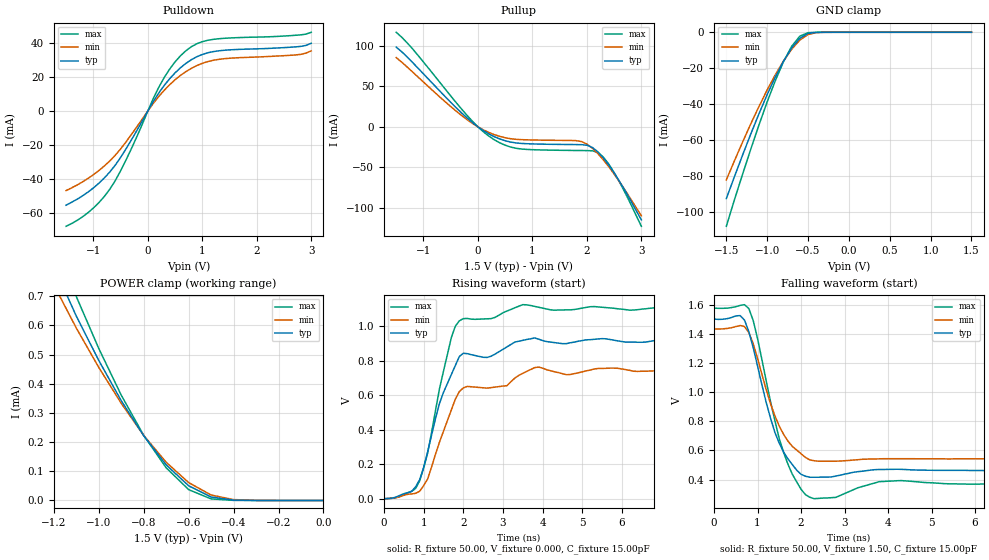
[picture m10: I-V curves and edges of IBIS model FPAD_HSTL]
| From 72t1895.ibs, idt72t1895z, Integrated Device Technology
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|   Model FPAD_HSTL
[Model]   FPAD_HSTL
Model_type   3-state
Polarity   Non-Inverting
Enable   Active-Low
Vmeas =  0.750V
C_comp   3.00pF   NA   NA
[Temperature Range]   25.00   85.00   -40.00
[Voltage Range]   1.50V   1.40V   1.60V
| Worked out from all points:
|   slope of the pulldown table from 0 to 0.225 V, typ, clamps not added: 19.3 ohm
|   slope of the pullup table from 0 to 0.225 V, typ, clamps not added: 23.5 ohm
|   GND clamp passes 1 mA (typ) near -0.51 V on its own axis
|   POWER clamp passes 1 mA (typ) near -1.28 V on its own axis
|   rising waveform, R_fixture 50.00, V_fixture 0.000, C_fixture 15.00pF: 20-80 % time 714ps typ, 695ps min, 594ps max; typ from 0 V to 0.911 V
|   falling waveform, R_fixture 50.00, V_fixture 1.50, C_fixture 15.00pF: 20-80 % time 562ps typ, 605ps min, 548ps max; typ from 1.5 V to 0.463 V
[Pulldown]
| voltage   I(typ)   I(min)   I(max)
-1.5V     -55.54mA   -46.94mA   -68mA
-1.1V     -47.85mA   -39.79mA   -60mA
-900mV    -42.65mA   -35.17mA   -54.12mA
-700mV    -36.05mA   -29.51mA   -46.23mA
-400mV    -22.33mA   -18.22mA   -28.88mA
200mV     10.57mA    8.525mA    13.92mA
400mV     19.01mA    15.49mA    24.67mA
700mV     28.12mA    23.26mA    35.58mA
900mV     32.02mA    26.81mA    39.69mA
1.2V      35.04mA    29.92mA    42.26mA
2.7V      37.81mA    33.05mA    44.66mA
3V        39.96mA    35.49mA    46.45mA
[Pullup]
| voltage   I(typ)   I(min)   I(max)
-1.5V     98.65mA    85.67mA    117mA
-1.2V     79.68mA    67.93mA    96.54mA
-300mV    17.26mA    14.08mA    22.02mA
0V        0A         0A         0A
300mV     -12.12mA   -9.576mA   -15.95mA
800mV     -20.5mA    -15.8mA    -27.4mA
1.9V      -22.02mA   -18.14mA   -29.27mA
2.1V      -25.42mA   -26.39mA   -29.62mA
2.2V      -30.83mA   -32.98mA   -31.59mA
2.3V      -38.24mA   -40.65mA   -37.27mA
2.5V      -56.93mA   -58.35mA   -56.49mA
3V        -115mA     -110mA     -123mA
[GND_clamp]
| voltage   I(typ)   I(min)   I(max)
-1.5V     -92.56mA   -82.16mA   -108mA
-1.4V     -80.26mA   -71.45mA   -93.09mA
-1.2V     -56.53mA   -50.9mA    -64.94mA
-1.1V     -45.3mA    -41.22mA   -51.5mA
-1V       -34.68mA   -32.07mA   -38.72mA
-900mV    -24.85mA   -23.59mA   -26.87mA
-800mV    -16.08mA   -15.96mA   -16.35mA
-700mV    -8.721mA   -9.411mA   -7.76mA
-600mV    -3.357mA   -4.326mA   -2.135mA
-500mV    -667uA     -1.241mA   -218uA
-400mV    -58.99uA   -179uA     -9.374uA
1.5V      15.04nA    17.39nA    15nA
[POWER_clamp]
| voltage   I(typ)   I(min)   I(max)
-1.5V     2.847mA    1.929mA    4.371mA
-1.2V     803uA      739uA      910uA
-1.1V     632uA      591uA      699uA
-1V       480uA      456uA      521uA
-900mV    342uA      333uA      361uA
-800mV    222uA      223uA      223uA
-700mV    122uA      131uA      112uA
-600mV    50.34uA    61.26uA    37.18uA
-500mV    11.87uA    18.7uA     5.404uA
-400mV    1.358uA    3.086uA    373nA
0V        15.04nA    15.59nA    16nA
[Ramp]
| variable   typ   min   max
dV/dt_r   0.55/0.30n   0.45/0.33n   0.67/0.31n
dV/dt_f   0.63/0.21n   0.55/0.23n   0.73/0.21n
R_load = 50.00
[Rising Waveform]
R_fixture = 50.00
V_fixture = 0.000
C_fixture = 15.00pF
R_dut = 0.75
L_dut = 8.10nH
C_dut = 0.53pF
| time   V(typ)   V(min)   V(max)
0s        0V         0V         0V
900ps     110mV      43.26mV    103mV
1.1ns     270mV      113mV      263mV
1.4ns     552mV      328mV      637mV
1.7ns     720mV      515mV      935mV
2ns       843mV      642mV      1.044V
2.6ns     819mV      641mV      1.043V
3.1ns     880mV      655mV      1.088V
3.9ns     925mV      763mV      1.11V
9.9ns     911mV      747mV      1.099V
[Falling Waveform]
R_fixture = 50.00
V_fixture = 1.50
C_fixture = 15.00pF
R_dut = 0.75
L_dut = 8.10nH
C_dut = 0.53pF
| time   V(typ)   V(min)   V(max)
0s        1.5V       1.433V     1.575V
600ps     1.524V     1.456V     1.594V
800ps     1.413V     1.407V     1.572V
1ns       1.178V     1.23V      1.366V
1.2ns     927mV      1.015V     1.074V
1.5ns     649mV      766mV      678mV
1.8ns     503mV      627mV      436mV
2.2ns     416mV      535mV      279mV
4.2ns     471mV      543mV      392mV
9.9ns     463mV      542mV      373mV
